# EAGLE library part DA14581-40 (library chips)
A better version of the DA14580 - faster boot
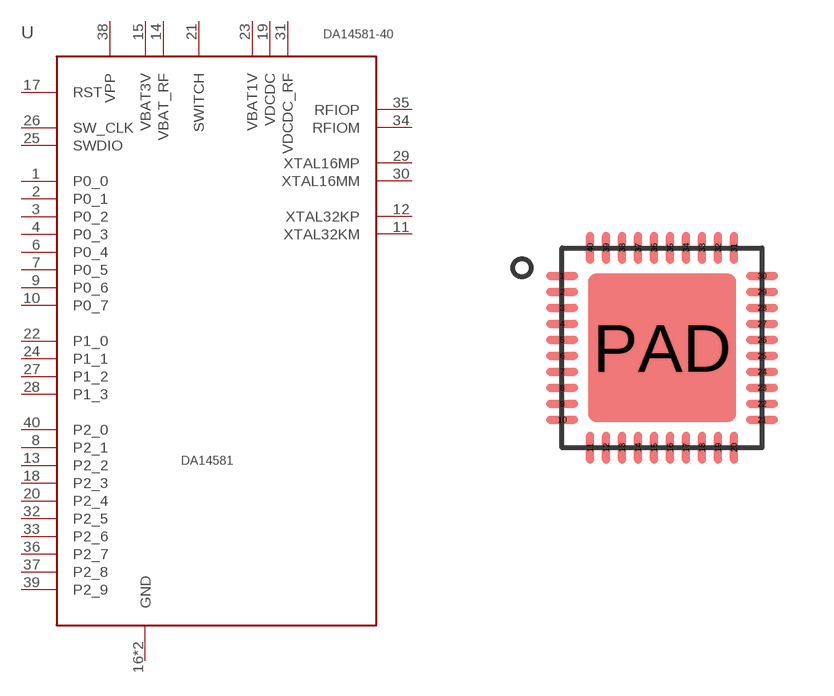
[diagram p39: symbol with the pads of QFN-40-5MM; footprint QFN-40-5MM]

Designator prefix -

## DA14581-40 (DIGIKEY: 1564-1016-1-ND)  [QFN-40-5MM]
1  P0_0
2  P0_1
3  P0_2
4  P0_3
6  P0_4
7  P0_5
8  P2_1
9  P0_6
10  P0_7
11  XTAL32KM
12  XTAL32KP
13  P2_2
14  VBAT_RF
15  VBAT3V
16  GND
17  RST
18  P2_3
19  VDCDC
20  P2_4
21  SWITCH
22  P1_0
23  VBAT1V
24  P1_1
25  SWDIO
26  SW_CLK
27  P1_2
28  P1_3
29  XTAL16MP
30  XTAL16MM
31  VDCDC_RF
32  P2_5
33  P2_6
34  RFIOM
35  RFIOP
36  P2_7
37  P2_8
38  VPP
39  P2_9
40  P2_0
PAD  GND

## Footprint QFN-40-5MM (pad centres in mm)
smd 0.8 x 0.2: 1 -2.5,1.8; 2 -2.5,1.4; 3 -2.5,1; 4 -2.5,0.6; 5 -2.5,0.2; 6 -2.5,-0.2; 7 -2.5,-0.6; 8 -2.5,-1; 9 -2.5,-1.4; 10 -2.5,-1.8; 21 2.5,-1.8; 22 2.5,-1.4; 23 2.5,-1; 24 2.5,-0.6; 25 2.5,-0.2; 26 2.5,0.2; 27 2.5,0.6; 28 2.5,1; 29 2.5,1.4; 30 2.5,1.8
smd 0.2 x 0.8: 11 -1.8,-2.5; 12 -1.4,-2.5; 13 -1,-2.5; 14 -0.6,-2.5; 15 -0.2,-2.5; 16 0.2,-2.5; 17 0.6,-2.5; 18 1,-2.5; 19 1.4,-2.5; 20 1.8,-2.5; 31 1.8,2.5; 32 1.4,2.5; 33 1,2.5; 34 0.6,2.5; 35 0.2,2.5; 36 -0.2,2.5; 37 -0.6,2.5; 38 -1,2.5; 39 -1.4,2.5; 40 -1.8,2.5
smd 3.7 x 3.7: PAD 0,0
